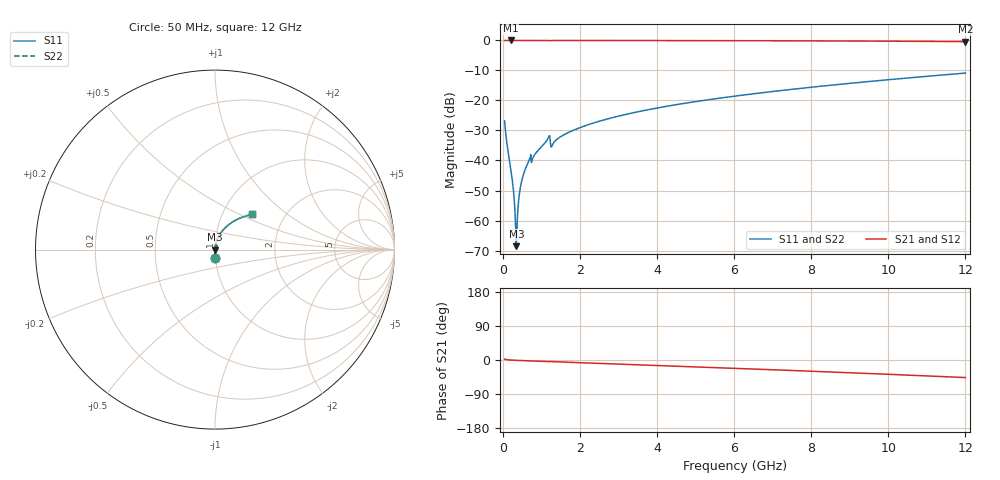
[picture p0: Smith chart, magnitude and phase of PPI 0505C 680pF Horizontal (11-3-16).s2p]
# MHz S MA R 50
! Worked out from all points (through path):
!   1601 points, 50 MHz to 12 GHz, reference 50 ohm
!   highest |S21| = 0.00 dB at 206.8 MHz (marker M1); lowest = -0.4 dB at 12 GHz (marker M2)
!   group delay of S21, straight-line fit = 10.7 ps
!   lowest |S11| = -68.5 dB at 356.2 MHz (marker M3), VSWR 1.00, Z = 50 + j0.011 ohm
!   |S11| at or under -10 dB: start of sweep to end of sweep
!   |S22| runs from -68.5 to -10.9 dB; largest |S21 - S12| = 0
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50  0.04578 -87.3  0.9988 2.5  0.9988 2.5  0.04578 -87.3
206.8438  0.007441 -87.8  0.9997 -0.1  0.9997 -0.1  0.007441 -87.8
259.125  0.004186 -86.1  0.9997 -0.4  0.9997 -0.4  0.004186 -86.1
311.4062  0.001709 -79.3  0.9996 -0.7  0.9996 -0.7  0.001709 -79.3
333.8125  0.0008249 -65.9  0.9996 -0.8  0.9996 -0.8  0.0008249 -65.9
356.2188  0.0003738 17.2  0.9996 -0.9  0.9996 -0.9  0.0003738 17.2
393.5625  0.001493 74.6  0.9996 -1.1  0.9996 -1.1  0.001493 74.6
445.8438  0.003165 81.7  0.9996 -1.3  0.9996 -1.3  0.003165 81.7
490.6562  0.004501 83.4  0.9996 -1.5  0.9996 -1.5  0.004501 83.4
565.3438  0.006595 84.5  0.9995 -1.8  0.9995 -1.8  0.006595 84.5
677.375  0.009773 84.6  0.9994 -2.3  0.9994 -2.3  0.009773 84.6
804.3438  0.01176 84.6  0.9993 -2.7  0.9993 -2.7  0.01176 84.6
1170.312  0.023 80.8  0.9977 -4.3  0.9977 -4.3  0.023 80.8
1304.75  0.01898 80.6  0.9981 -4.4  0.9981 -4.4  0.01898 80.6
1536.281  0.02567 83.1  0.9989 -5.4  0.9989 -5.4  0.02567 83.1
2044.156  0.03604 81.6  0.9985 -7.3  0.9985 -7.3  0.03604 81.6
2903.062  0.05289 78.8  0.9976 -10.4  0.9976 -10.4  0.05289 78.8
4038.312  0.07559 74.8  0.996 -14.5  0.996 -14.5  0.07559 74.8
6025  0.1182 67.5  0.9915 -22.0  0.9915 -22.0  0.1182 67.5
8019.156  0.1665 59.9  0.9843 -29.7  0.9843 -29.7  0.1665 59.9
10013.31  0.2221 51.8  0.9729 -37.8  0.9729 -37.8  0.2221 51.8
12000  0.286 43.3  0.9557 -46.4  0.9557 -46.4  0.286 43.3
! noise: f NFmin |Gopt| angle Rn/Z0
50  0.0003131  0.8342  0.1703  0.0003989
1372  0.003651  0.6494  3.367  0.001976
2701  0.004749  0.5134  6.2  0.001696
4031  0.006358  0.4733  8.922  0.002037
5360  0.007894  0.4473  11.48  0.00236
6682  0.009396  0.4303  13.88  0.002682
8012  0.01092  0.4196  16.16  0.003024
9341  0.01249  0.4142  18.36  0.003398
1.067e+04  0.01414  0.4135  20.49  0.00382
1.2e+04  0.01589  0.417  22.59  0.004305
